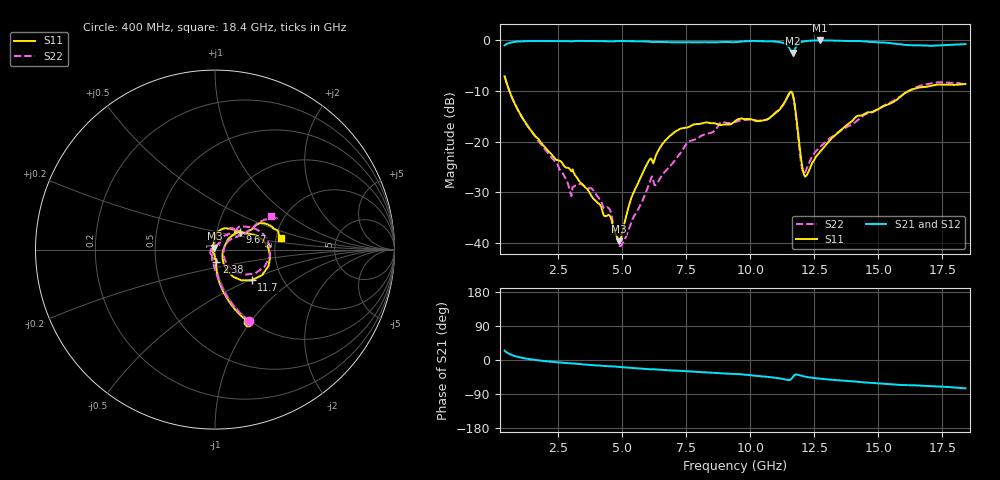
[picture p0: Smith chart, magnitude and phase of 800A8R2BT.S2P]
!  American Technical Ceramics  Date:  12/17/08
!  One Norden Lane
!  Huntington Station,  NY.  11746-2102
!  Tel:  (631) 622-4700  Fax:  (631) 622-4748
!  Part Number  800A8R2BT
!  Description: Broardband capacitor  Mounting Orientation: Vertical
!  Application:
# GHZ S DB R 50
! Freq  |S11|  S11 Ph  |S21|  S21 Ph  |S12|  S12 Ph  |S22|  S22 Ph
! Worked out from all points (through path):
!   401 points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, 400 MHz to 18.4 GHz, reference 50 ohm
!   highest |S21| = -0.02 dB at 12.73 GHz (marker M1); lowest = -2.5 dB at 11.65 GHz (marker M2)
!   group delay of S21, straight-line fit = 12.4 ps
!   lowest |S11| = -39.7 dB at 4.855 GHz (marker M3), VSWR 1.02, Z = 49.6 + j0.957 ohm
!   |S11| at or under -10 dB: 586.8 MHz to 16.19 GHz (15.6 GHz wide, 186 % of centre)
!   |S22| runs from -40.7 to -7.1 dB; largest |S21 - S12| = 0.0024
!   S11 on the Smith chart (normalised r, x): 400 MHz: 0.97, -0.97; 2.38 GHz: 1.01, -0.14; 9.67 GHz: 1.29, +0.26; 11.7 GHz: 1.41, -0.52; 18.4 GHz: 2.12, +0.31
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0.4  -7.10 -65.4  -0.98 24.6  -0.98 24.6  -7.10 -64.5
1.165  -15.87 -83.8  -0.17 4.5  -0.17 4.5  -15.93 -84.1
2.38  -23.42 -83.3  -0.13 -5.6  -0.13 -5.6  -23.98 -102.2
2.965  -25.57 -88.0  -0.19 -8.8  -0.19 -8.8  -30.06 -117.8
3.415  -28.35 -91.5  -0.11 -11.3  -0.11 -11.3  -28.42 -117.5
4.495  -34.54 -157.0  -0.20 -16.6  -0.21 -16.6  -33.31 170.7
4.855  -39.70 111.3  -0.12 -18.1  -0.11 -18.1  -40.19 121.1
5.485  -29.56 103.6  -0.18 -21.4  -0.18 -21.4  -34.50 76.7
6.07  -23.53 87.7  -0.26 -24.5  -0.26 -24.5  -28.04 60.4
6.43  -21.55 87.0  -0.31 -25.6  -0.31 -25.6  -27.65 54.1
7.6  -17.12 56.7  -0.36 -30.0  -0.36 -30.0  -19.97 52.6
9.4  -15.99 40.6  -0.36 -37.0  -0.36 -37.0  -16.16 45.8
9.67  -15.45 34.8  -0.21 -37.9  -0.21 -37.9  -15.78 44.4
11.29  -12.67 20.8  -0.52 -50.1  -0.52 -50.2  -12.61 32.0
11.65  -10.50 -28.4  -2.47 -45.6  -2.47 -45.6  -10.69 -19.0
11.695  -11.46 -39.8  -2.27 -41.4  -2.26 -41.4  -11.71 -30.6
12.055  -25.76 -36.4  -0.23 -42.8  -0.23 -42.8  -26.09 -16.8
12.415  -24.24 23.0  -0.06 -46.9  -0.05 -46.9  -22.91 28.1
12.73  -21.95 33.9  -0.02 -49.3  -0.02 -49.4  -21.03 32.2
14.125  -15.10 34.8  -0.11 -57.0  -0.11 -57.1  -16.05 30.9
15.43  -12.54 28.9  -0.53 -64.1  -0.52 -64.1  -12.33 29.8
18.4  -8.61 9.7  -0.74 -74.8  -0.73 -74.9  -8.70 31.1
